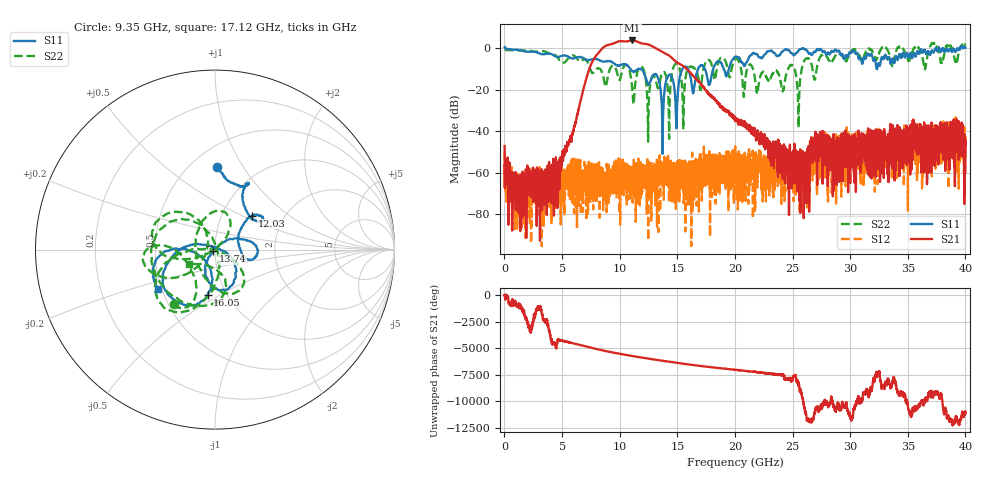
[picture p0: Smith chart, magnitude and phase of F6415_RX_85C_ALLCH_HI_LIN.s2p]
!Keysight Technologies,N5245B,MY52451815,A.15.70.20
!Date: Wednesday, April 17, 2024 16:15:27
!Correction: S33(C  2-Port  )
!S43(C  2-Port  )
!S34(C  2-Port  )
!S44(C  2-Port  )
!S2P File: Measurements: S33, S43, S34, S44:
# Hz S  RI  R 50
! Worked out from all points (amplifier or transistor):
!   4000 points, 10 MHz to 40 GHz, reference 50 ohm
!   highest |S21| = 3.8 dB at 11.1 GHz (marker M1)
!   |S21| within 3 dB of that: 8.669 GHz to 12.89 GHz (4.219 GHz wide, 39.1 % of centre)
!   unconditionally stable (mu >= 1): 99.54 MHz to 25.86 GHz; 25.94 GHz to 32.71 GHz; 34.53 GHz to 35.53 GHz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
!   at 6.67 GHz: K = 6171.27, MAG = -20.5 dB, |S12| = -64.5 dB
!   at 20.01 GHz: K = 5632.82, MAG = -30.2 dB, |S12| = -54.5 dB
!   at 40 GHz: K = 2785.05, MSG = -6.5 dB, |S12| = -46.8 dB
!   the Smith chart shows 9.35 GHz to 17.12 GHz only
!   S11 on the Smith chart (normalised r, x): 9.35 GHz: 0.66, +0.78; 12.03 GHz: 1.38, +0.57; 13.74 GHz: 0.98, -0.02; 16.05 GHz: 0.82, -0.44; 17.12 GHz: 0.48, -0.24
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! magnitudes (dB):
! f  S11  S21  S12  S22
! 10 MHz  0.4  -47.2  -49.9  -0.9
! 1.18 GHz  -0.8  -64.2  -73.1  -1.1
! 4.46 GHz  -4.0  -52.6  -60.5  -3.5
! 6.68 GHz  -4.4  -23.7  -62.7  -6.1
! 9.35 GHz  -6.7  2.1  -63.1  -8.4
! 11.1 GHz  -11.1  3.8  -67.0  -20.2
! 12.03 GHz  -11.1  2.2  -65.3  -9.8
! 12.46 GHz  -17.4  1.9  -67.0  -45.1
! 13.34 GHz  -14.5  -0.6  -59.4  -19.3
! 13.74 GHz  -38.8  -1.9  -64.0  -11.8
! 14.99 GHz  -26.6  -6.9  -54.6  -7.6
! 15.53 GHz  -9.2  -8.7  -62.0  -33.7
! 16.05 GHz  -11.9  -11.3  -75.3  -9.0
! 17.12 GHz  -8.3  -17.7  -63.4  -15.6
! 20.01 GHz  -4.1  -33.8  -54.5  -5.4
! 21.94 GHz  -3.0  -40.1  -59.8  -21.4
! 24.95 GHz  -2.4  -53.4  -53.7  -8.3
! 25.5 GHz  -1.2  -54.8  -50.5  -32.9
! 26.67 GHz  -3.2  -43.8  -48.9  -8.6
! 33.34 GHz  -4.3  -64.6  -46.5  -1.9
! 39.3 GHz  -0.2  -39.3  -40.4  -5.5
! 40 GHz  0.2  -59.8  -46.8  1.6
